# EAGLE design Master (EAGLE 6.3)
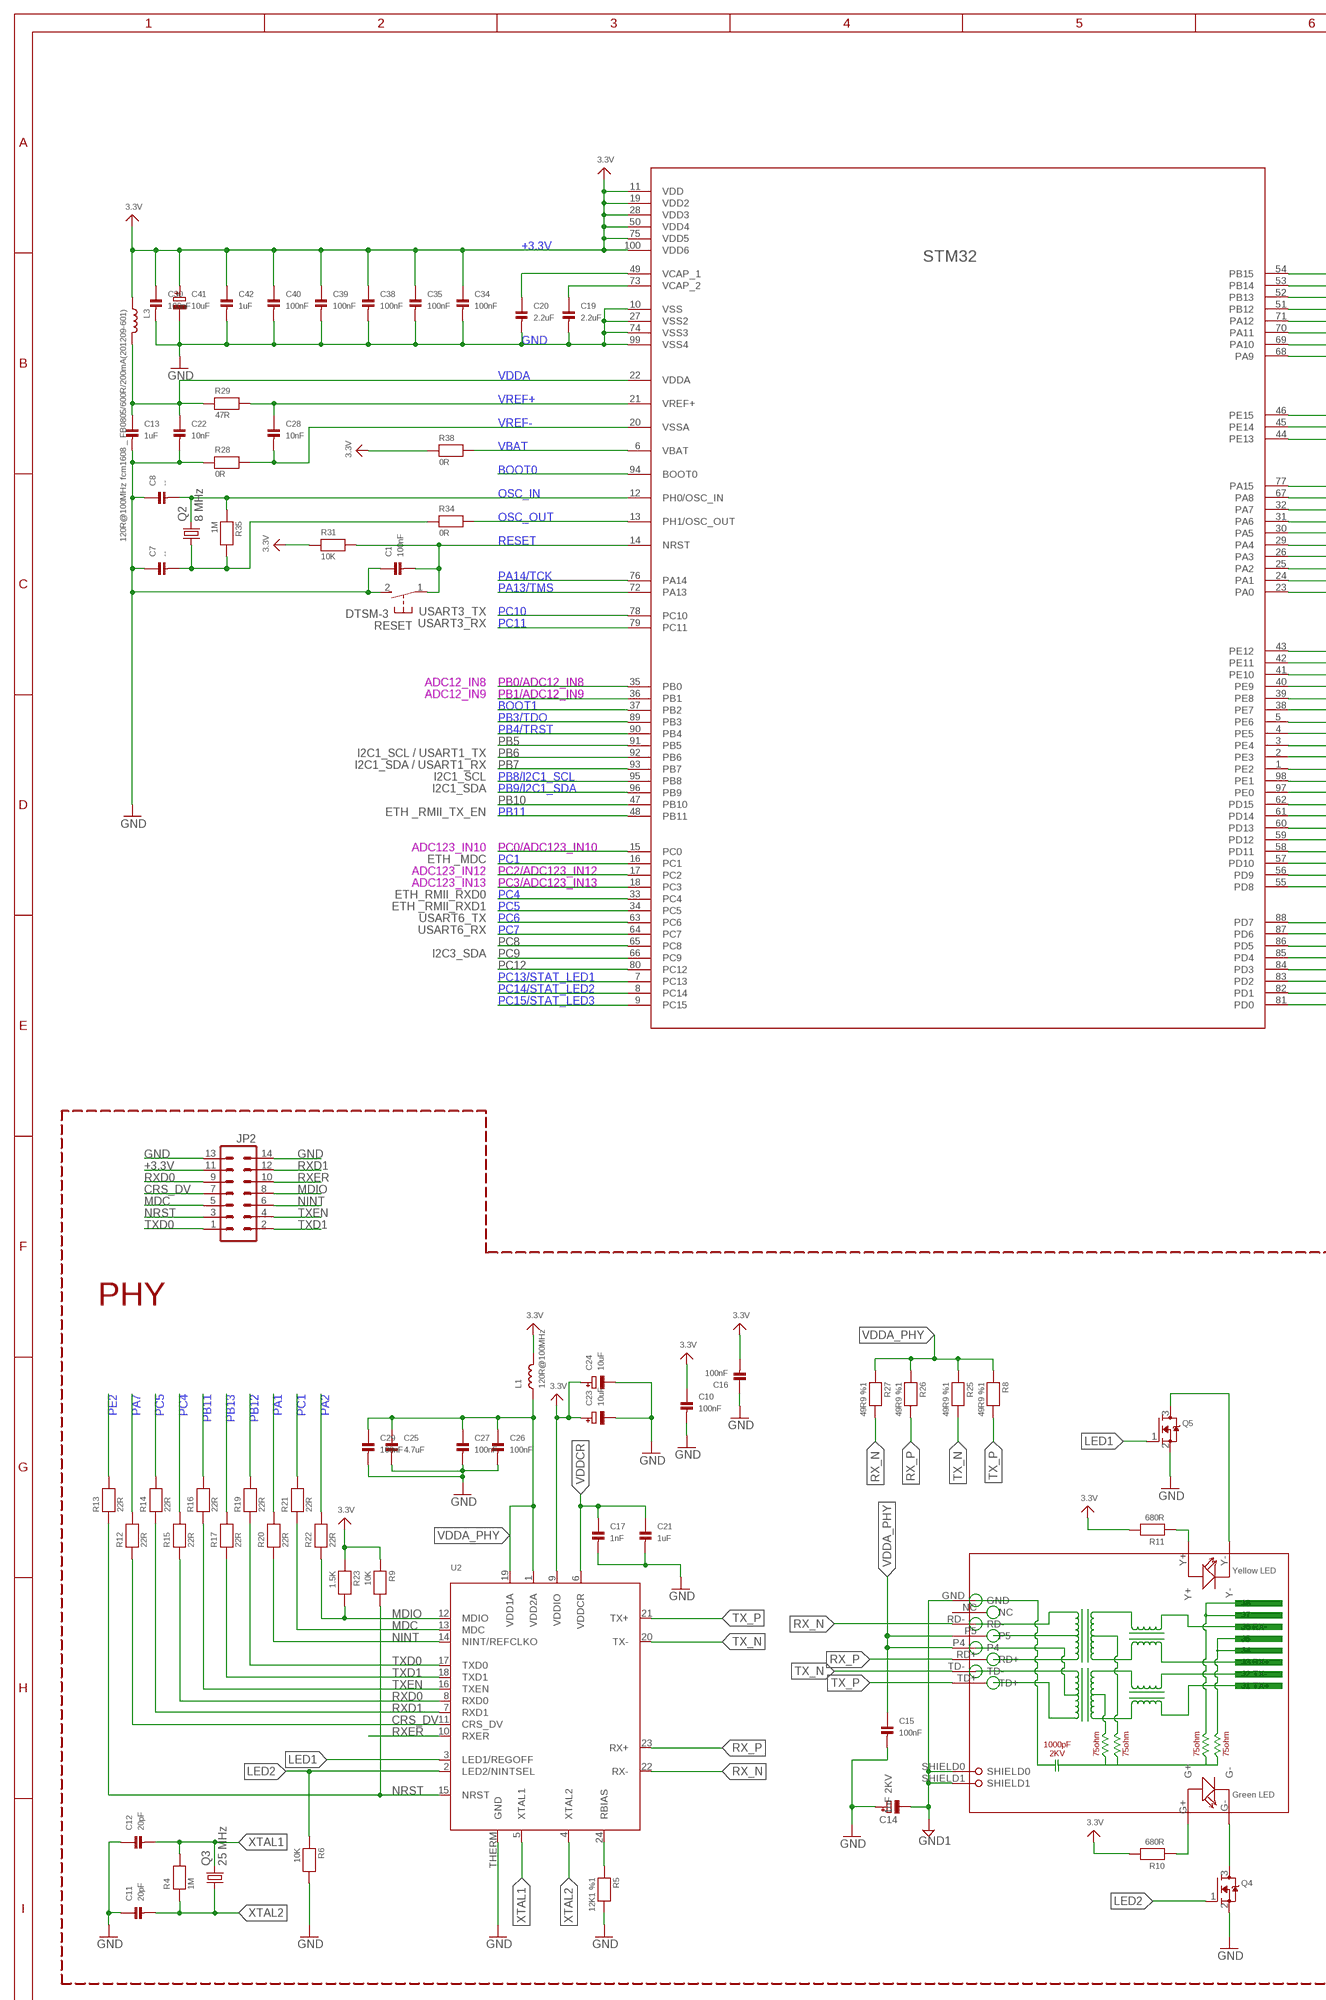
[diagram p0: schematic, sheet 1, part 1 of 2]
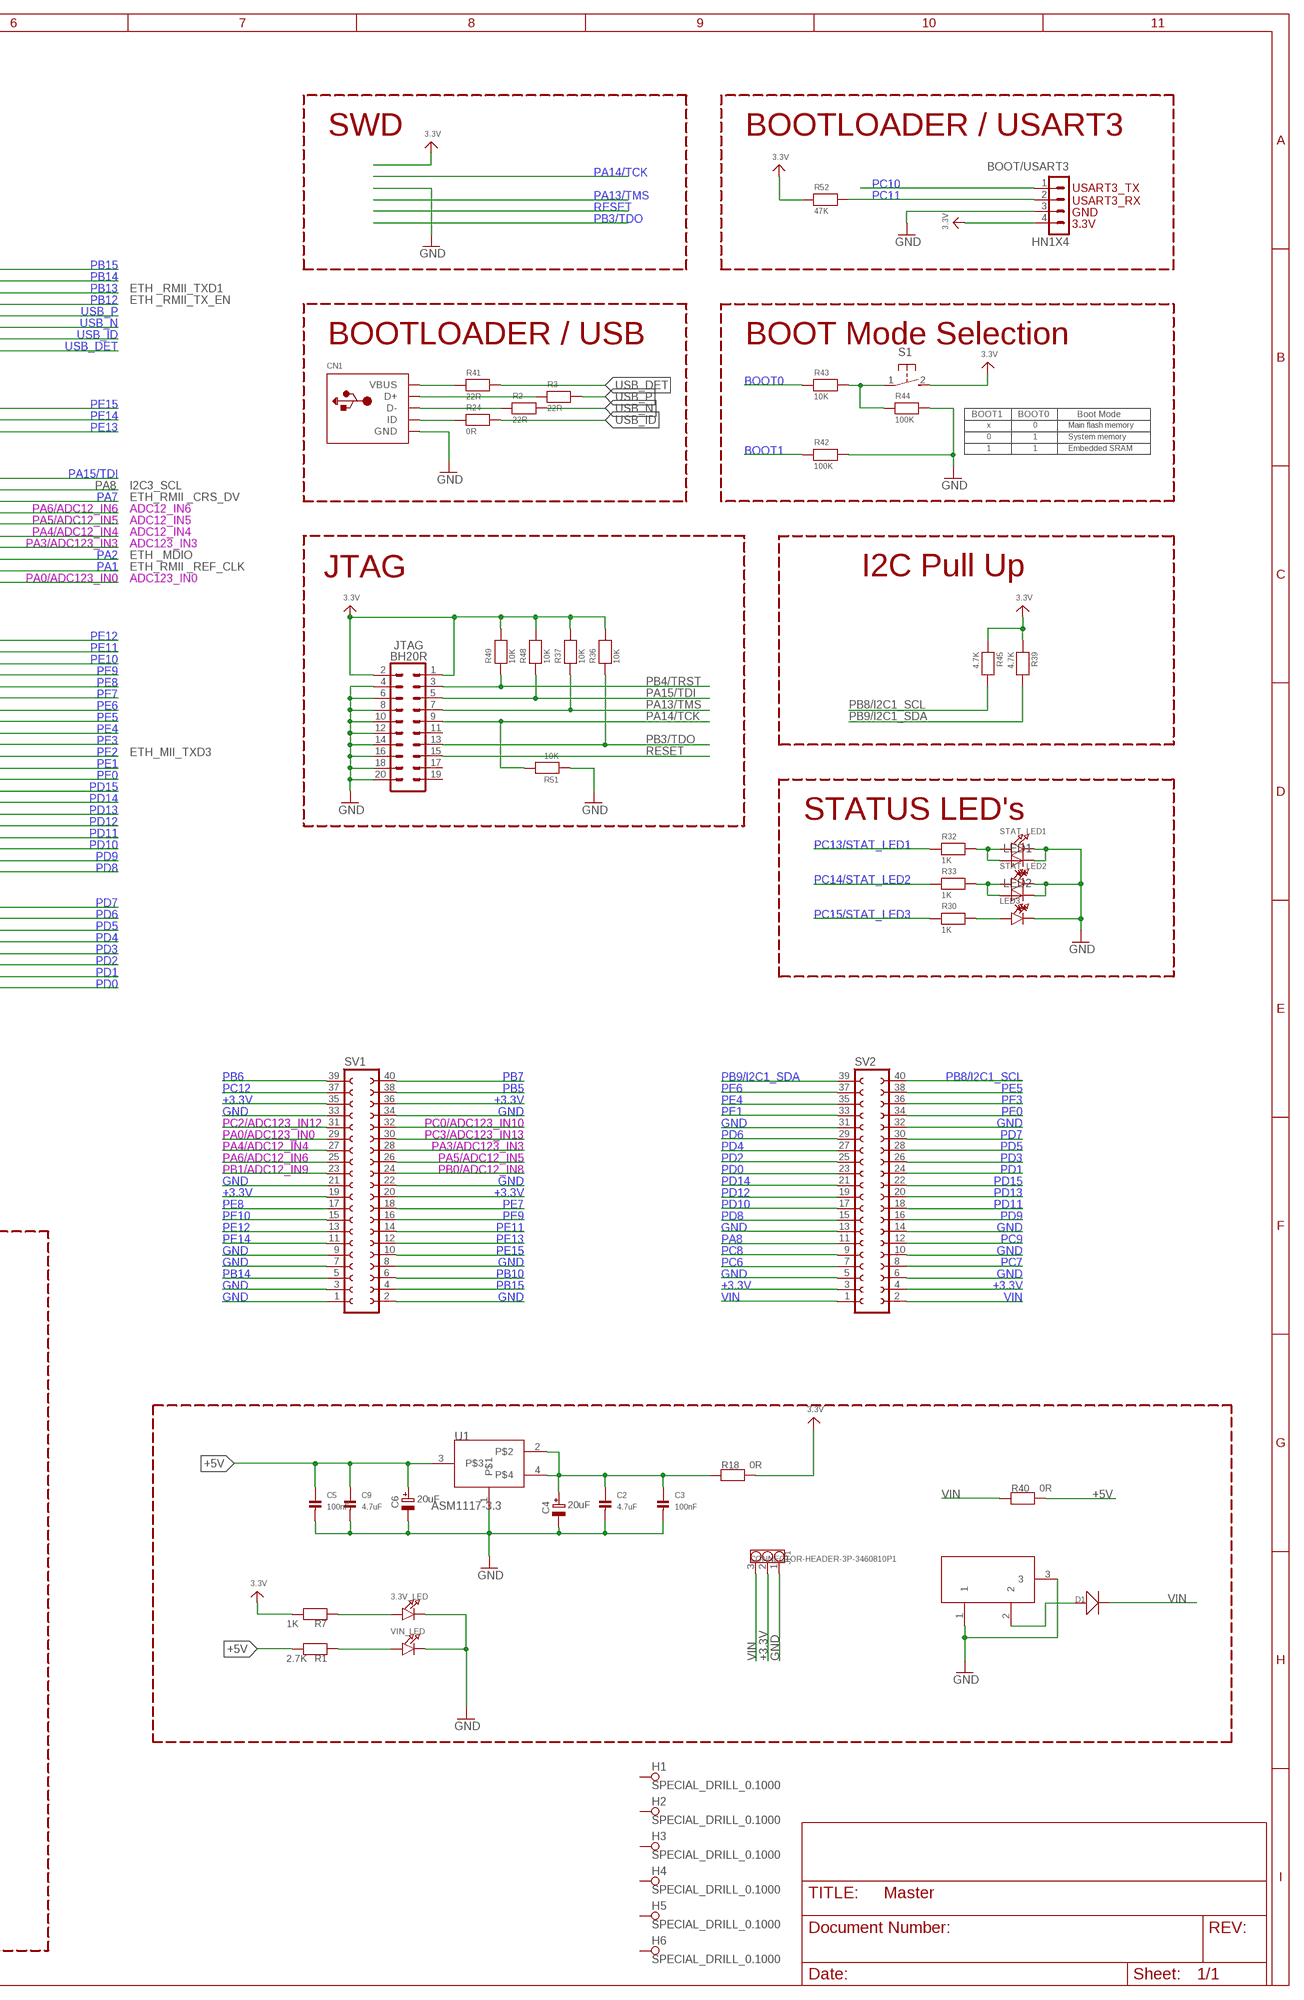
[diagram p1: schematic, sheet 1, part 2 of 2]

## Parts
3.3V_LED  LED0805  [CHIPLED_0805]
BOOT/USART3  HN1X4  CON4HN1X4  [HN1X4]
C1  100nF  CAP_CERAMIC_0603  [_0603]
C2  4.7uF  CAP_CERAMIC0805  [0805]
C3  100nF  CAP_CERAMIC0805  [0805]
C4  20uF  CAP_TANTALUMB/3528_REFLOW  [EIA3528-21/B-R]
C5  100nF  CAP_CERAMIC0805  [0805]
C6  20uF  CAP_TANTALUMB/3528_REFLOW  [EIA3528-21/B-R]
C7  --  CAP_CERAMIC_0603  [_0603]
C8  --  CAP_CERAMIC_0603  [_0603]
C9  4.7uF  CAP_CERAMIC0805  [0805]
C10  100nF  CAP_CERAMIC_0603  [_0603]
C11  20pF  CAP_CERAMIC_0603  [_0603]
C12  20pF  CAP_CERAMIC_0603  [_0603]
C13  1uF  CAP_CERAMIC_0805  [_0805]
C14  1nF 2KV  CAP_TANTALUMB/3528_REFLOW  [EIA3528-21/B-R]
C15  100nF  CAP_CERAMIC_0805  [_0805]
C16  100nF  CAP_CERAMIC_0603  [_0603]
C17  1nF  CAP_CERAMIC_0603  [_0603]
C19  2.2uF  CAP_CERAMIC1206  [1206]
C20  2.2uF  CAP_CERAMIC1206  [1206]
C21  1uF  CAP_CERAMIC_0805  [_0805]
C22  10nF  CAP_CERAMIC_0603  [_0603]
C23  10uF  CAP_TANTALUMB/3528_REFLOW  [EIA3528-21/B-R]
C24  10uF  CAP_TANTALUMB/3528_REFLOW  [EIA3528-21/B-R]
C25  4.7uF  CAP_CERAMIC_0805  [_0805]
C26  100nF  CAP_CERAMIC_0603  [_0603]
C27  100nF  CAP_CERAMIC_0603  [_0603]
C28  10nF  CAP_CERAMIC_0603  [_0603]
C29  100nF  CAP_CERAMIC_0603  [_0603]
C30  100nF  CAP_CERAMIC_0603  [_0603]
C34  100nF  CAP_CERAMIC_0603  [_0603]
C35  100nF  CAP_CERAMIC_0603  [_0603]
C38  100nF  CAP_CERAMIC_0603  [_0603]
C39  100nF  CAP_CERAMIC_0603  [_0603]
C40  100nF  CAP_CERAMIC_0603  [_0603]
C41  10uF  CAP_TANTALUMB/3528_REFLOW  [EIA3528-21/B-R]
C42  1uF  CAP_CERAMIC_0805  [_0805]
CN1  USBMINIBLARGE  [USB-MINIB_LARGER]
D1  D-D1206  [LL-34]
H1  SPECIAL_DRILL_0.1000  [PAD_0.1000]
H2  SPECIAL_DRILL_0.1000  [PAD_0.1000]
H3  SPECIAL_DRILL_0.1000  [PAD_0.1000]
H4  SPECIAL_DRILL_0.1000  [PAD_0.1000]
H5  SPECIAL_DRILL_0.1000  [PAD_0.1000]
H6  SPECIAL_DRILL_0.1000  [PAD_0.1000]
JP1  CONNECTOR-HEADER-3P-3460810P1  [1X3P-2.54-2.54-11.6-3.0-BLACK-MALE]
JP2  MA07-2  [MA07-2]
JTAG  BH20R  ML20R  [BH20R]
L1  120R@100MHz  INDUCTOR_0805  [_0805]
L3  120R@100MHz fcm1608 _ FB0805/600R/200mA(201209-601)  INDUCTOR_0805  [_0805]
LED1  LED5MM  [LED5MM]
LED2  LED5MM  [LED5MM]
LED3  LED0805  [CHIPLED_0805]
Q2  8 MHz  CRYSTALHC49UP  [HC49UP]
Q3  25 MHz  CRYSTALHC49UP  [HC49UP]
Q4  MOSFET-NWIDE  [SOT23-WIDE]
Q5  MOSFET-NWIDE  [SOT23-WIDE]
R1  2.7K  RESISTOR_0603  [_0603]
R2  22R  RESISTOR_0603  [_0603]
R3  22R  RESISTOR_0603  [_0603]
R4  1M  RESISTOR_0603  [_0603]
R5  12K1 %1  RESISTOR_0603  [_0603]
R6  10K  RESISTOR_0603  [_0603]
R7  1K  RESISTOR_0603  [_0603]
R8  49R9 %1  RESISTOR_0603  [_0603]
R9  10K  RESISTOR_0603  [_0603]
R10  680R  RESISTOR_0805  [_0805]
R11  680R  RESISTOR_0805  [_0805]
R12  22R  RESISTOR_0603  [_0603]
R13  22R  RESISTOR_0603  [_0603]
R14  22R  RESISTOR_0603  [_0603]
R15  22R  RESISTOR_0603  [_0603]
R16  22R  RESISTOR_0603  [_0603]
R17  22R  RESISTOR_0603  [_0603]
R18  0R  RESISTOR0805  [0805]
R19  22R  RESISTOR_0603  [_0603]
R20  22R  RESISTOR_0603  [_0603]
R21  22R  RESISTOR_0603  [_0603]
R22  22R  RESISTOR_0603  [_0603]
R23  1.5K  RESISTOR_0603  [_0603]
R24  0R  RESISTOR_0603  [_0603]
R25  49R9 %1  RESISTOR_0603  [_0603]
R26  49R9 %1  RESISTOR_0603  [_0603]
R27  49R9 %1  RESISTOR_0603  [_0603]
R28  0R  RESISTOR_0603  [_0603]
R29  47R  RESISTOR_0603  [_0603]
R30  1K  RESISTOR_0603  [_0603]
R31  10K  RESISTOR_0603  [_0603]
R32  1K  RESISTOR_0603  [_0603]
R33  1K  RESISTOR_0603  [_0603]
R34  0R  RESISTOR_0603  [_0603]
R35  1M  RESISTOR_0603  [_0603]
R36  10K  RESISTOR_0603  [_0603]
R37  10K  RESISTOR_0603  [_0603]
R38  0R  RESISTOR_0603  [_0603]
R39  4.7K  RESISTOR1206  [1206]
R40  0R  RESISTOR0805  [0805]
R41  22R  RESISTOR_0603  [_0603]
R42  100K  RESISTOR_0603  [_0603]
R43  10K  RESISTOR_0603  [_0603]
R44  100K  RESISTOR_0603  [_0603]
R45  4.7K  RESISTOR1206  [1206]
R48  10K  RESISTOR_0603  [_0603]
R49  10K  RESISTOR_0603  [_0603]
R51  10K  RESISTOR_0603  [_0603]
R52  47K  RESISTOR_0603  [_0603]
RESET  DTSM-3  [DTSM-3]
RJ1  HR911105A  [HR911105A]
S1  31-XX  [B3F-31XX]
STAT_LED1  LED0805  [CHIPLED_0805]
STAT_LED2  LED0805  [CHIPLED_0805]
STM32  STM32F407  [100LQFP]
SV1  FE20-2  [FE20-2]
SV2  FE20-2  [FE20-2]
U1  ASM1117-3.3  [SOT223]
U2  LAN8720  [QFN24_4MM]
VIN_LED  LED0805  [CHIPLED_0805]
X1  DC21MMX  [DC-21MM]

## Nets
+3.3V: BOOT/USART3.4 C10.1 C16.2 C23.+ C24.+ C30.1 C34.1 C35.1 C38.1 C39.1 C40.1 C41.+ C42.1 JP1.2 JP2.11 JTAG.1 JTAG.2 L1.2 L3.1 R7.2 R9.1 R10.2 R11.2 R18.2 R23.1 R31.1 R36.2 R37.2 R38.1 R39.1 R45.1 R48.2 R49.2 R52.1 S1.2(S) STM32.11(VDD) STM32.19(VDD2) STM32.28(VDD3) STM32.50(VDD4) STM32.75(VDD5) STM32.100(VDD6) SV1.19 SV1.20 SV1.35 SV1.36 SV2.3 SV2.4 U2.9(VDDIO) ; supply symbol labelled 3.3V
+5V: C5.1 C6.+ C9.1 R1.2 R40.2 U1.3
BOOT0: R43.1 STM32.94(BOOT0)
BOOT1: R42.1 STM32.37(PB2)
CRS_DV: JP2.7 R12.1 U2.11(CRS_DV)
GND: 3.3V_LED.C BOOT/USART3.3 C1.1 C2.2 C3.2 C4.- C5.2 C6.- C7.1 C8.1 C9.2 C10.2 C11.1 C12.1 C13.2 C14.+ C15.2 C16.1 C17.2 C19.2 C20.2 C21.2 C22.2 C23.- C24.- C25.2 C26.2 C27.2 C29.2 C30.2 C34.2 C35.2 C38.2 C39.2 C40.2 C41.- C42.2 CN1.GND JP1.1 JP2.13 JP2.14 JTAG.4 JTAG.6 JTAG.8 JTAG.10 JTAG.12 JTAG.14 JTAG.16 JTAG.18 JTAG.20 LED1.K(C) LED2.K(C) LED3.C Q4.2(S) Q5.2(S) R5.2 R6.2 R28.1 R42.2 R44.2 R51.1 RESET.2 STAT_LED1.C STAT_LED2.C STM32.10(VSS) STM32.27(VSS2) STM32.74(VSS3) STM32.99(VSS4) SV1.1 SV1.2 SV1.3 SV1.7 SV1.8 SV1.9 SV1.21 SV1.22 SV1.33 SV1.34 SV2.5 SV2.6 SV2.10 SV2.13 SV2.14 SV2.31 SV2.32 U1.1 U2.THERM(GND) VIN_LED.C X1.1 X1.3
GND1: C14.- RJ1.GND RJ1.SHIELD0 RJ1.SHIELD1
LED1: Q5.1(G) U2.3(LED1/REGOFF)
LED2: Q4.1(G) R6.1 U2.2(LED2/NINTSEL)
MDC: JP2.5 R21.1 U2.13(MDC)
MDIO: JP2.8 R22.1 R23.2 U2.12(MDIO)
N$1: LED1.A R32.2 STAT_LED1.A
N$2: LED2.A R33.2 STAT_LED2.A
N$3: CN1.VBUS R41.1
N$4: LED3.A R30.2
N$5: D1.A(+) X1.2
N$6: C2.1 C3.1 C4.+ R18.1 U1.2 U1.4
N$7: 3.3V_LED.A R7.1
N$8: R43.2 R44.1 S1.1(P)
N$9: CN1.ID R24.1
N$10: R1.1 VIN_LED.A
N$11: CN1.D+ R3.1
N$12: R5.1 U2.24(RBIAS)
N$13: R10.1 RJ1.G+
N$14: R11.1 RJ1.Y+
N$27: Q4.3(D) RJ1.G-
N$28: Q5.3(D) RJ1.Y-
N$29: CN1.D- R2.1
N$35: C19.1 STM32.73(VCAP_2)
N$36: C20.1 STM32.49(VCAP_1)
N$45: C7.2 Q2.1 R34.1 R35.2
NINT: JP2.6 R20.1 U2.14(NINT/REFCLKO)
NRST: JP2.3 R9.2 R13.1 U2.15(NRST)
OSC_IN: C8.2 Q2.2 R35.1 STM32.12(PH0/OSC_IN)
OSC_OUT: R34.2 STM32.13(PH1/OSC_OUT)
PA0/ADC123_IN0: STM32.23(PA0) SV1.29
PA1: R20.2 STM32.24(PA1)
PA2: R22.2 STM32.25(PA2)
PA3/ADC123_IN3: STM32.26(PA3) SV1.28
PA4/ADC12_IN4: STM32.29(PA4) SV1.27
PA5/ADC12_IN5: STM32.30(PA5) SV1.26
PA6/ADC12_IN6: STM32.31(PA6) SV1.25
PA7: R12.2 STM32.32(PA7)
PA8: STM32.67(PA8) SV2.11
PA13/TMS: JTAG.7 R37.1 STM32.72(PA13)
PA14/TCK: JTAG.9 R51.2 STM32.76(PA14)
PA15/TDI: JTAG.5 R48.1 STM32.77(PA15)
PB0/ADC12_IN8: STM32.35(PB0) SV1.24
PB1/ADC12_IN9: STM32.36(PB1) SV1.23
PB3/TDO: JTAG.13 R36.1 STM32.89(PB3)
PB4/TRST: JTAG.3 R49.1 STM32.90(PB4)
PB5: STM32.91(PB5) SV1.38
PB6: STM32.92(PB6) SV1.39
PB7: STM32.93(PB7) SV1.40
PB8/I2C1_SCL: R45.2 STM32.95(PB8) SV2.40
PB9/I2C1_SDA: R39.2 STM32.96(PB9) SV2.39
PB10: STM32.47(PB10) SV1.6
PB11: R16.2 STM32.48(PB11)
PB12: R19.2 STM32.51(PB12)
PB13: R17.2 STM32.52(PB13)
PB14: STM32.53(PB14) SV1.5
PB15: STM32.54(PB15) SV1.4
PC0/ADC123_IN10: STM32.15(PC0) SV1.32
PC1: R21.2 STM32.16(PC1)
PC2/ADC123_IN12: STM32.17(PC2) SV1.31
PC3/ADC123_IN13: STM32.18(PC3) SV1.30
PC4: R15.2 STM32.33(PC4)
PC5: R14.2 STM32.34(PC5)
PC6: STM32.63(PC6) SV2.7
PC7: STM32.64(PC7) SV2.8
PC8: STM32.65(PC8) SV2.9
PC9: STM32.66(PC9) SV2.12
PC10: BOOT/USART3.1 STM32.78(PC10)
PC11: BOOT/USART3.2 R52.2 STM32.79(PC11)
PC12: STM32.80(PC12) SV1.37
PC13/STAT_LED1: R32.1 STM32.7(PC13)
PC14/STAT_LED2: R33.1 STM32.8(PC14)
PC15/STAT_LED3: R30.1 STM32.9(PC15)
PD0: STM32.81(PD0) SV2.23
PD1: STM32.82(PD1) SV2.24
PD2: STM32.83(PD2) SV2.25
PD3: STM32.84(PD3) SV2.26
PD4: STM32.85(PD4) SV2.27
PD5: STM32.86(PD5) SV2.28
PD6: STM32.87(PD6) SV2.29
PD7: STM32.88(PD7) SV2.30
PD8: STM32.55(PD8) SV2.15
PD9: STM32.56(PD9) SV2.16
PD10: STM32.57(PD10) SV2.17
PD11: STM32.58(PD11) SV2.18
PD12: STM32.59(PD12) SV2.19
PD13: STM32.60(PD13) SV2.20
PD14: STM32.61(PD14) SV2.21
PD15: STM32.62(PD15) SV2.22
PE0: STM32.97(PE0) SV2.34
PE1: STM32.98(PE1) SV2.33
PE2: R13.2 STM32.1(PE2)
PE3: STM32.2(PE3) SV2.36
PE4: STM32.3(PE4) SV2.35
PE5: STM32.4(PE5) SV2.38
PE6: STM32.5(PE6) SV2.37
PE7: STM32.38(PE7) SV1.18
PE8: STM32.39(PE8) SV1.17
PE9: STM32.40(PE9) SV1.16
PE10: STM32.41(PE10) SV1.15
PE11: STM32.42(PE11) SV1.14
PE12: STM32.43(PE12) SV1.13
PE13: STM32.44(PE13) SV1.12
PE14: STM32.45(PE14) SV1.11
PE15: STM32.46(PE15) SV1.10
RESET: C1.2 JTAG.15 R31.2 RESET.1 STM32.14(NRST)
RX_N: R27.2 RJ1.RD- U2.22(RX-)
RX_P: R26.2 RJ1.RD+ U2.23(RX+)
RXD0: JP2.9 R15.1 U2.8(RXD0)
RXD1: JP2.12 R14.1 U2.7(RXD1)
RXER: JP2.10 U2.10(RXER)
TX_N: R25.2 RJ1.TD- U2.20(TX-)
TX_P: R8.2 RJ1.TD+ U2.21(TX+)
TXD0: JP2.1 R19.1 U2.17(TXD0)
TXD1: JP2.2 R17.1 U2.18(TXD1)
TXEN: JP2.4 R16.1 U2.16(TXEN)
USB_DET: R41.2 STM32.68(PA9)
USB_ID: R24.2 STM32.69(PA10)
USB_N: R2.2 STM32.70(PA11)
USB_P: R3.2 STM32.71(PA12)
VBAT: R38.2 STM32.6(VBAT)
VDDA: C13.1 C22.1 L3.2 R29.1 STM32.22(VDDA)
VDDA_PHY: C15.1 C25.1 C26.1 C27.1 C29.1 L1.1 R8.1 R25.1 R26.1 R27.1 RJ1.P4 RJ1.P5 U2.1(VDD2A) U2.19(VDD1A)
VDDCR: C17.1 C21.1 U2.6(VDDCR)
VIN: D1.C(-) JP1.3 R40.1 SV2.1 SV2.2
VREF+: C28.1 R29.2 STM32.21(VREF+)
VREF-: C28.2 R28.2 STM32.20(VSSA)
XTAL1: C12.2 Q3.2 R4.2 U2.5(XTAL1)
XTAL2: C11.2 Q3.1 R4.1 U2.4(XTAL2)
Unconnected: H1.1 H2.1 H3.1 H4.1 H5.1 H6.1 JTAG.11 JTAG.17 JTAG.19 RJ1.NC

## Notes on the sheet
- SWD | BOOTLOADER / USART3
- USART3_TX
- USART3_RX
- GND
- 3.3V
- ETH _RMII_TXD1
- ETH _RMII_TX_EN
- BOOTLOADER / USB | BOOT Mode Selection
- BOOT1 | BOOT0 | Boot Mode
- x | 0 | Main flash memory
- 0 | 1 | System memory
- 1 | 1 | Embedded SRAM
- I2C3_SCL
- ETH_RMII _CRS_DV
- ADC12_IN6
- ADC12_IN5
- ADC12_IN4
- ADC123_IN3
- ETH _MDIO
- ETH_RMII _REF_CLK
- JTAG | I2C Pull Up
- ADC123_IN0
- USART3_TX
- USART3_RX
- ADC12_IN8
- ADC12_IN9
- I2C1_SCL / USART1_TX
- I2C1_SDA / USART1_RX | ETH_MII_TXD3
- I2C1_SCL
- I2C1_SDA
- ETH _RMII_TX_EN
- STATUS LED's
- ADC123_IN10
- ETH _MDC
- ADC123_IN12
- ADC123_IN13
- ETH_RMII_RXD0
- ETH _RMII_RXD1
- USART6_TX
- USART6_RX
- I2C3_SDA
- PHY

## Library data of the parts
3.3V_LED LED3 STAT_LED1 STAT_LED2 VIN_LED = microbuilder:LED: LED
BOOT/USART3 = Penko:CON4
C1-C3 C5 C7-C13 C15-C17 C19-C22 C25-C30 C34 C35 C38-C40 C42 = microbuilder:CAP_CERAMIC: Ceramic Capacitors
C4 C6 C14 C23 C24 C41 = microbuilder:CAP_TANTALUM: Tantalum Capacitors
CN1 = microbuilder:USB: USB Connectors USBMINIB - Surface Mount Female Mini-B USB Connector 4UConnector: 06564
D1 = OPL Eagle Library:D*: DIODE
H1-H6 = special-drill:SPECIAL_DRILL_: Special drills
JP1 = OPL Eagle Library:CONNECTOR-HEADER-3P
JP2 = con-lstb:MA07-2: PIN HEADER; OC_FARNELL: unknown; OC_NEWARK: unknown
JTAG = con-harting-ml:ML20: HARTING
L1 L3 = microbuilder:INDUCTOR: Inductors
LED1 LED2 = led:LED: LED
Q2 Q3 = crystal:CRYSTAL: CRYSTAL; OC_FARNELL: unknown; OC_NEWARK: unknown
Q4 Q5 = microbuilder:MOSFET-N: N-Channel Mosfet LEGEND VDS: Voltage Drain-Source ID: Drain Current RDS(ON): Drain-Source On-State Resistance VGS(TH): Gate-Source Threshold Voltage CISS: Drain-Source Input Capacitance SOT-23 Name VDS ID RDS(ON) VGS(TH) CISS Order Number 2N7002E 60V 260mA 2.5 Ohm 2.5V @ 250uA 26.7pF @ 25V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
R1-R45 R48 R49 R51 R52 = microbuilder:RESISTOR: Resistors
RESET = switch-tact:DTSM-3
RJ1 = Itead_BP_110825.lbr:HR911105A: SOC006
S1 = switch-omron:31-XX: OMRON SWITCH; MPN: B3F-3100; OC_FARNELL: 959704; OC_NEWARK: 36M3582
STM32 = BaseApp:STM32F407
SV1 SV2 = con-lsta:FE20-2: FEMALE HEADER; OC_FARNELL: unknown; OC_NEWARK: unknown
U1 = Itead_IC_110429:ASM1117-3.3: ICP006
U2 = microbuilder:LAN8720: LAN8720A 10/100 Ethernet PHY Mouser: 886-LAN8720AI-CP
X1 = powersupply:DC21MM

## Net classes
0 default: width 0.152 mm, drill 0.305 mm, clearance 0.152 mm

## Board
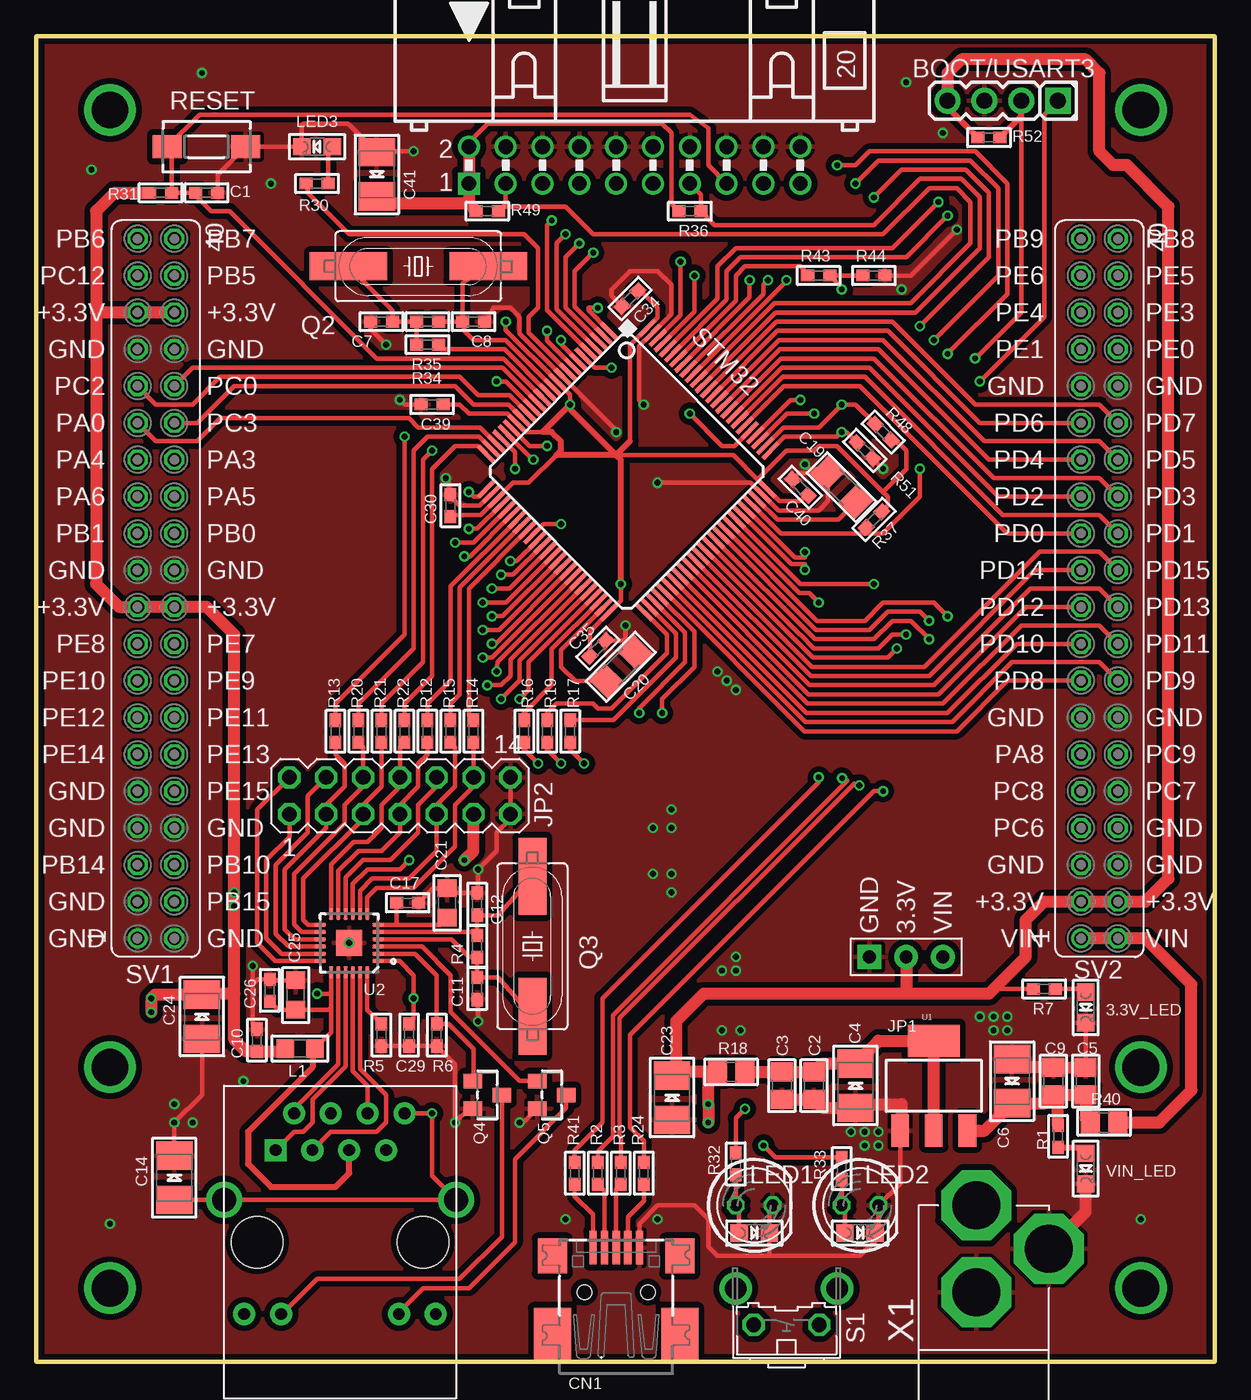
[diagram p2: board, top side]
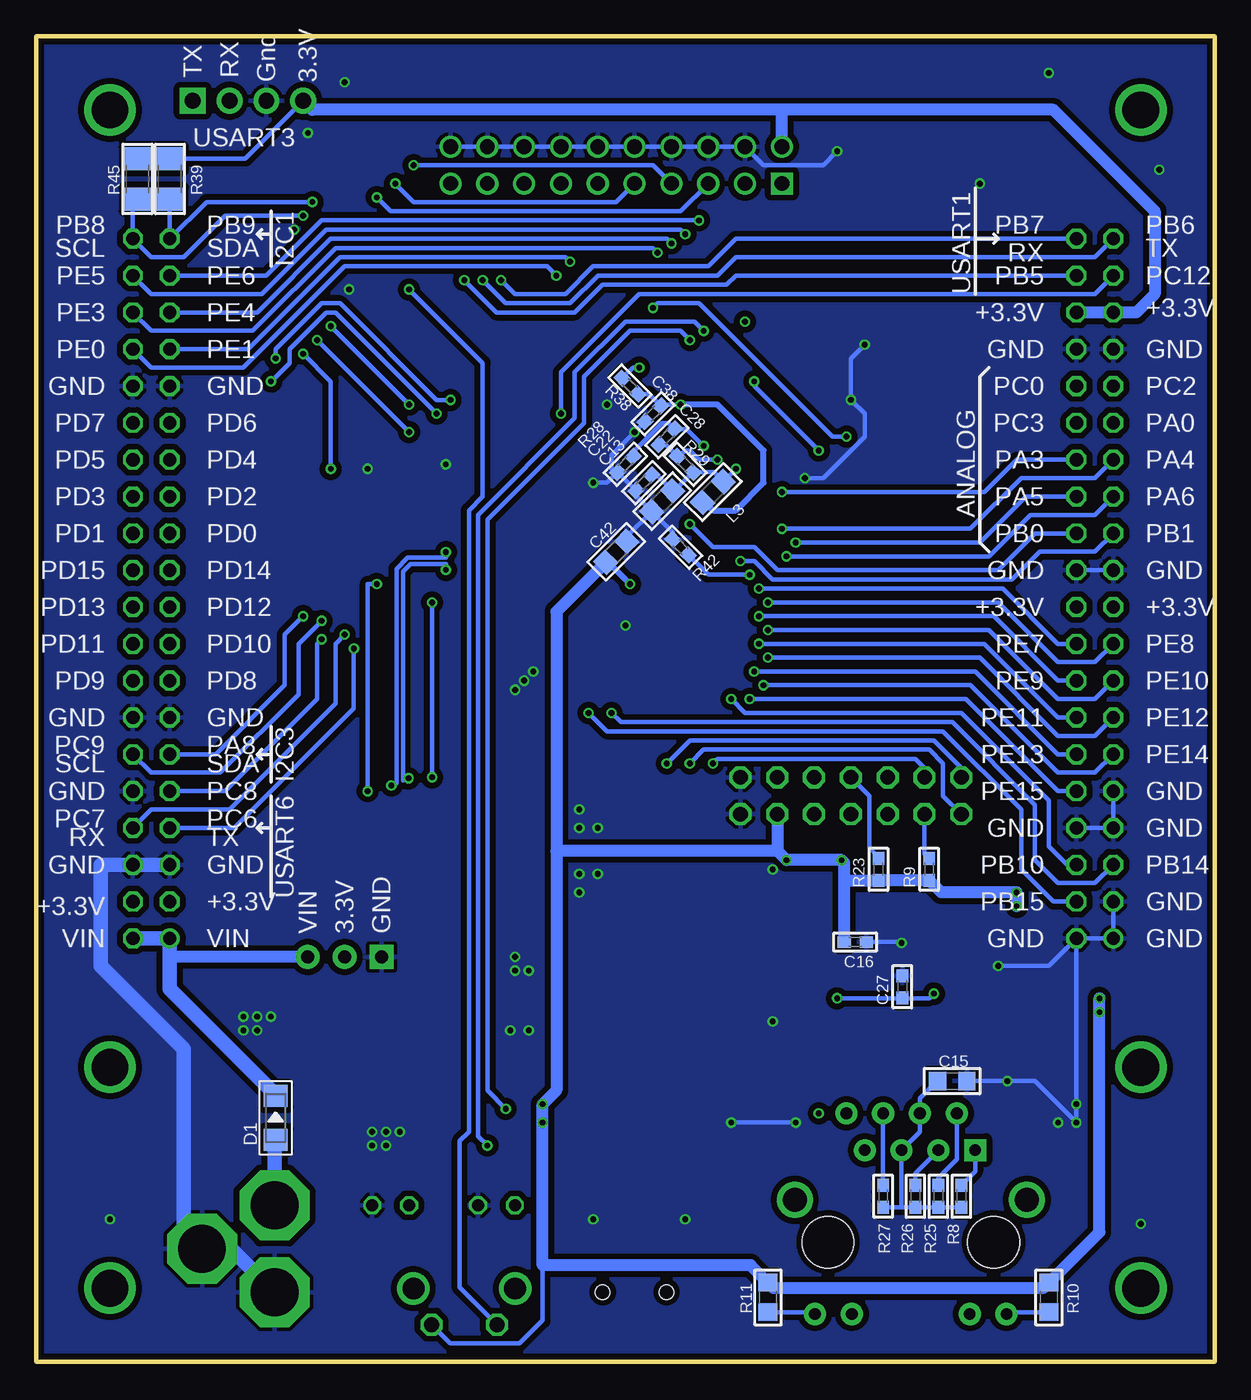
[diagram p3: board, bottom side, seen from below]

Size 81.28 x 91.44 mm. Coordinates in mm from the lower left corner, seen from the top.
Outline: 0,0 81.28,0 81.28,91.44 0,91.44 0,0
Copper layers (1*2*15*16): Top 0.035mm / dielectric 0.2mm / Route2 0.0175mm / dielectric 1.1mm / Route15 0.0175mm / dielectric 0.2mm / Bottom 0.035mm
Design rules "SeeedStudio_DRU_no_angle_20130527": minimum track width 6mil, minimum drill 12mil, track to track 6mil, track to pad 6mil, pad to pad 6mil, via to via 6mil, smd to smd 0mil, copper to edge 10mil, drill to drill 10mil, minimum pad ring 6mil, minimum via ring 6mil, stop-mask expansion 2mil, vias tented up to drill 25mil, thermal gap 10mil

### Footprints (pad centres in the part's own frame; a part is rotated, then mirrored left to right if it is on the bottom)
CHIPLED_0805 = smd 1.2 x 1.2: A 0,-1.05; C 0,1.05
HN1X4 = drill 1.1 pad 1.778 square: 1 -3.81,0 | drill 1.1 pad 1.778: 2 -1.27,0; 3 1.27,0; 4 3.81,0
_0603 = smd 0.9 x 0.8: 1 -0.762,0; 2 0.762,0
0805 = smd 1.3 x 1.5: 1 -0.95,0; 2 0.95,0
EIA3528-21/B-R = smd 1.95 x 2.5: + 1.525,0; - -1.525,0
_0805 = smd 1.2 x 1.3: 1 -1.016,0; 2 1.016,0
1206 = smd 1.6 x 1.8: 1 -1.4,0; 2 1.4,0
USB-MINIB_LARGER = smd 0.5 x 2.308: D+ 0,4.064; D- -0.8,4.064; GND 1.6,4.064; ID 0.8,4.064; VBUS -1.6,4.064 | smd 2.54 x 3.81: GND1 -4.4,-2; GND4 4.4,-2 | smd 2 x 2.4: GND2 -4.4,3.5; GND3 4.4,3.5 | hole 1: -2.2,1; 2.2,1
LL-34 = smd 1.524 x 1.676: A -1.524,0; C 1.524,0
PAD_0.1000 = drill 2.54 pad 2.54: 1 0,0
1X3P-2.54-2.54-11.6-3.0-BLACK-MALE = drill 0.889 pad 1.651 square: 1 0,2.54 | drill 0.889 pad 1.651: 2 0,0; 3 0,-2.54
MA07-2 = drill 1.016 octagon: 1 -7.62,-1.27; 2 -7.62,1.27; 3 -5.08,-1.27; 4 -5.08,1.27; 5 -2.54,-1.27; 6 -2.54,1.27; 7 0,-1.27; 8 0,1.27; 9 2.54,-1.27; 10 2.54,1.27; 11 5.08,-1.27; 12 5.08,1.27; 13 7.62,-1.27; 14 7.62,1.27
BH20R = drill 1.016 square: 1 -11.43,-1.27 | drill 1.016: 2 -11.43,1.27; 3 -8.89,-1.27; 4 -8.89,1.27; 5 -6.35,-1.27; 6 -6.35,1.27; 7 -3.81,-1.27; 8 -3.81,1.27; 9 -1.27,-1.27; 10 -1.27,1.27; 11 1.27,-1.27; 12 1.27,1.27; 13 3.81,-1.27; 14 3.81,1.27; 15 6.35,-1.27; 16 6.35,1.27; 17 8.89,-1.27; 18 8.89,1.27; 19 11.43,-1.27; 20 11.43,1.27
LED5MM = drill 0.813 octagon: A -1.27,0; K 1.27,0
HC49UP = smd 5.334 x 1.93: 1 -4.826,0; 2 4.826,0
SOT23-WIDE = smd 1 x 1.27: 1 -0.95,-1; 2 0.95,-1; 3 0,1
DTSM-3 = smd 2 x 1.6: 1 -2.7,0; 2 2.7,0
HR911105A = drill 0.813 pad 1.524: G+ 4.953,-6.604; G- 4.953,-4.064; GND -8.89,4.445; NC -6.35,3.175; P4 -8.89,-0.635; P5 -6.35,0.635; RD+ -6.35,-1.905; RD- -8.89,1.905; TD- -8.89,-3.175; Y+ 4.953,6.604; Y- 4.953,4.064 | drill 1.651 pad 2.159: SHIELD0 -2.921,8.001; SHIELD1 -2.921,-8.001 | drill 0.813 pad 1.524 square: TD+ -6.35,-4.445 | hole 3.556: 0,-5.715; 0,5.715
B3F-31XX = drill 1.016 octagon: 1 -2.261,-1.245; 2 2.261,-1.245 | drill 1.499 pad 2.159: 3 -3.505,1.245; 4 3.505,1.245
100LQFP = smd 1.5 x 0.3: 1 -6.18,9.08; 2 -6.18,8.58; 3 -6.18,8.08; 4 -6.18,7.58; 5 -6.18,7.08; 6 -6.18,6.58; 7 -6.18,6.08; 8 -6.18,5.58; 9 -6.18,5.08; 10 -6.18,4.58; 11 -6.18,4.08; 12 -6.18,3.58; 13 -6.18,3.08; 14 -6.18,2.58; 15 -6.18,2.08; 16 -6.18,1.58; 17 -6.18,1.08; 18 -6.18,0.58; 19 -6.18,0.08; 20 -6.18,-0.42; 21 -6.18,-0.92; 22 -6.18,-1.42; 23 -6.18,-1.92; 24 -6.18,-2.42; 25 -6.18,-2.92; 51 9.26,-2.92; 52 9.26,-2.42; 53 9.26,-1.92; 54 9.26,-1.42; 55 9.26,-0.92; 56 9.26,-0.42; 57 9.26,0.08; 58 9.26,0.58; 59 9.26,1.08; 60 9.26,1.58; 61 9.26,2.08; 62 9.26,2.58; 63 9.26,3.08; 64 9.26,3.58; 65 9.26,4.08; 66 9.26,4.58; 67 9.26,5.08; 68 9.26,5.58; 69 9.26,6.08; 70 9.26,6.58; 71 9.26,7.08; 72 9.26,7.58; 73 9.26,8.08; 74 9.26,8.58; 75 9.26,9.08 | smd 0.3 x 1.5: 26 -4.46,-4.64; 27 -3.96,-4.64; 28 -3.46,-4.64; 29 -2.96,-4.64; 30 -2.46,-4.64; 31 -1.96,-4.64; 32 -1.46,-4.64; 33 -0.96,-4.64; 34 -0.46,-4.64; 35 0.04,-4.64; 36 0.54,-4.64; 37 1.04,-4.64; 38 1.54,-4.64; 39 2.04,-4.64; 40 2.54,-4.64; 41 3.04,-4.64; 42 3.54,-4.64; 43 4.04,-4.64; 44 4.54,-4.64; 45 5.04,-4.64; 46 5.54,-4.64; 47 6.04,-4.64; 48 6.54,-4.64; 49 7.04,-4.64; 50 7.54,-4.64; 76 7.54,11.1; 77 7.04,11.1; 78 6.54,11.1; 79 6.04,11.1; 80 5.54,11.1; 81 5.04,11.1; 82 4.54,11.1; 83 4.04,11.1; 84 3.54,11.1; 85 3.04,11.1; 86 2.54,11.1; 87 2.04,11.1; 88 1.54,11.1; 89 1.04,11.1; 90 0.54,11.1; 91 0.04,11.1; 92 -0.46,11.1; 93 -0.96,11.1; 94 -1.46,11.1; 95 -1.96,11.1; 96 -2.46,11.1; 97 -2.96,11.1; 98 -3.46,11.1; 99 -3.96,11.1; 100 -4.46,11.1
FE20-2 = drill 0.914: 1 -24.13,1.27 | drill 0.914 octagon: 2 -24.13,-1.27; 3 -21.59,1.27; 4 -21.59,-1.27; 5 -19.05,1.27; 6 -19.05,-1.27; 7 -16.51,1.27; 8 -16.51,-1.27; 9 -13.97,1.27; 10 -13.97,-1.27; 11 -11.43,1.27; 12 -11.43,-1.27; 13 -8.89,1.27; 14 -8.89,-1.27; 15 -6.35,1.27; 16 -6.35,-1.27; 17 -3.81,1.27; 18 -3.81,-1.27; 19 -1.27,1.27; 20 -1.27,-1.27; 21 1.27,1.27; 22 1.27,-1.27; 23 3.81,1.27; 24 3.81,-1.27; 25 6.35,1.27; 26 6.35,-1.27; 27 8.89,1.27; 28 8.89,-1.27; 29 11.43,1.27; 30 11.43,-1.27; 31 13.97,1.27; 32 13.97,-1.27; 33 16.51,1.27; 34 16.51,-1.27; 35 19.05,1.27; 36 19.05,-1.27; 37 21.59,1.27; 38 21.59,-1.27; 39 24.13,1.27; 40 24.13,-1.27
SOT223 = smd 1.219 x 2.235: 1 -2.311,-3.099; 2 0,-3.099; 3 2.311,-3.099 | smd 3.6 x 2.2: 4 0,3.099
QFN24_4MM = smd 0.8 x 0.28: 1 -2,1.25; 2 -2,0.75; 3 -2,0.25; 4 -2,-0.25; 5 -2,-0.75; 6 -2,-1.25; 13 2,-1.25; 14 2,-0.75; 15 2,-0.25; 16 2,0.25; 17 2,0.75; 18 2,1.25 | smd 0.28 x 0.8: 7 -1.25,-2; 8 -0.75,-2; 9 -0.25,-2; 10 0.25,-2; 11 0.75,-2; 12 1.25,-2; 19 1.25,2; 20 0.75,2; 21 0.25,2; 22 -0.25,2; 23 -0.75,2; 24 -1.25,2 | smd 1.778 x 1.778: THERM 0,0
DC-21MM = drill 3.302 pad 4.826 octagon: 1 -5.08,-3.353; 2 -0.076,-6.35; 3 -0.076,-0.356

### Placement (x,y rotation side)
3.3V_LED  72.39,24.45 180 top
BOOT/USART3  66.67,87 180 top
C1  11.75,80.64 180 top
C2  53.66,19.05 270 top
C3  51.44,19.05 270 top
C4  56.52,19.05 90 top
C5  72.39,19.37 90 top
C6  67.31,19.37 270 top
C7  23.81,71.75 0 top
C8  30.16,71.75 180 top
C9  70.17,19.37 90 top
C10  15.22,22.19 90 top
C11  30.41,25.75 90 top
C12  30.41,31.57 270 top
C13  38.1,59.37 225 bottom
C14  9.53,12.7 90 top
C15  18.1,19.37 0 bottom
C16  24.79,28.96 180 bottom
C17  25.62,31.67 0 top
C19  55.56,60.33 135 top
C20  40.32,47.94 45 top
C21  28.34,31.65 90 top
C22  39.37,60.64 225 bottom
C23  43.86,18.23 90 top
C24  11.43,23.81 90 top
C25  17.9,25.3 90 top
C26  16.11,25.62 90 top
C27  21.54,25.87 90 bottom
C28  37.78,63.82 45 bottom
C29  25.72,22.54 270 top
C30  28.57,59.05 90 top
C34  40.96,73.34 225 top
C35  38.73,49.21 45 top
C38  38.73,65.41 225 bottom
C39  27.3,66.04 180 top
C40  52.7,60.33 135 top
C41  23.5,81.92 270 top
C42  41.27,55.88 45 bottom
CN1  40.01,3.81 0 top
D1  64.77,16.83 90 bottom
H1  5.08,5.08 0 top
H2  76.2,5.08 0 top
H3  76.2,86.36 0 top
H4  5.08,86.36 0 top
H5  5.08,20.32 0 top
H6  76.2,20.32 0 top
JP1  60.01,27.94 90 top
JP2  25.08,39.05 0 top
JTAG  41.27,82.55 0 top
L1  18.19,21.61 180 top
L3  34.61,60.01 45 bottom
LED1  49.53,10.79 0 top
LED2  56.83,10.79 0 top
LED3  19.37,83.82 90 top
Q2  26.35,75.56 0 top
Q3  34.22,28.66 90 top
Q4  31.11,18.41 270 top
Q5  35.56,18.41 270 top
R1  70.48,15.56 90 top
R2  38.73,13.02 90 top
R3  40.32,13.02 90 top
R4  30.41,28.66 90 top
R5  23.81,22.54 270 top
R6  27.62,22.54 270 top
R7  69.53,25.72 180 top
R8  17.46,11.43 90 bottom
R9  19.68,33.97 90 bottom
R10  11.43,4.45 90 bottom
R11  30.8,4.45 90 bottom
R12  26.99,43.5 90 top
R13  20.64,43.5 90 top
R14  30.16,43.5 90 top
R15  28.57,43.5 90 top
R16  33.66,43.5 90 top
R17  36.83,43.5 90 top
R18  47.94,20 180 top
R19  35.24,43.5 90 top
R20  22.23,43.5 90 top
R21  23.81,43.5 90 top
R22  25.4,43.5 90 top
R23  23.18,33.97 90 bottom
R24  41.91,13.02 90 top
R25  19.05,11.43 90 bottom
R26  20.64,11.43 90 bottom
R27  22.86,11.43 90 bottom
R28  40.64,61.91 45 bottom
R29  36.51,61.91 135 bottom
R30  19.37,81.28 0 top
R31  8.57,80.64 0 top
R32  48.26,13.65 270 top
R33  55.56,13.34 270 top
R34  26.99,70.17 0 top
R35  26.99,71.75 180 top
R36  45.09,79.38 180 top
R37  57.78,58.1 45 top
R38  40.32,67.31 135 bottom
R39  72.07,81.6 270 bottom
R40  73.66,16.51 180 top
R41  37.15,13.02 90 top
R42  36.83,56.2 135 bottom
R43  53.98,74.93 0 top
R44  57.78,74.93 0 top
R45  74.3,81.6 270 bottom
R48  58.42,64.14 315 top
R49  31.11,79.38 180 top
R51  57.15,62.87 135 top
R52  65.72,84.45 0 top
RESET  11.75,83.82 0 top
RJ1  20.95,8.26 270 top
S1  51.75,3.81 0 top
STAT_LED1  49.53,8.89 270 top
STAT_LED2  56.83,8.89 270 top
STM32  37.47,60.33 315 top
SV1  8.26,53.34 90 top
SV2  73.34,53.34 90 top
U1  61.91,19.05 0 top
U2  21.59,28.89 180 top
VIN_LED  72.39,13.34 180 top
X1  64.77,4.45 180 top

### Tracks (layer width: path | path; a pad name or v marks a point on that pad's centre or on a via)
+3.3V  (via drill 0.4)
  Top 0.305: U2.9 21.84,32.95 22.86,33.97 25.08,33.97 v25.72,34.61 | R36.2 43.81,79.88 43.81,84.77 43.18,85.41 31.11,85.41 29.84,84.14 JTAG.2 | v32.38,71.75 32.38,71.17 STM32.11 36.83,66.73 v36.83,66.04 | 44.13,20.02 C23.+ | R7.2 66.36,25.72 66.2,25.88 | C35.1 38.2,50.39 STM32.50 40.32,52.52 v40.32,53.66 | C30.1 28.45,58.29 28.57,58.42 30.67,58.42 STM32.28 32.89,60.64 33.97,60.64 35.88,62.55 | C39.1 29.21,66.04 29.84,65.41 32.5,65.41 STM32.19 33.77,64.14 34.92,64.14 | C34.1 41.69,73.88 42.86,72.71 42.86,72.03 STM32.100 40.96,70.12 40.96,63.5 | C40.1 53.24,59.91 52.7,59.37 51.26,59.37 STM32.75 49.76,60.87 | R37.2 58.74,59.05 58.74,59.69 58.42,60.01 | 58.42,60.01 55.24,63.18 53.98,63.18 53.66,62.87 51.75,62.87 49.76,60.87 | R48.2 59.59,63.28 60.01,62.87 60.01,61.59 58.42,60.01 | 49.76,60.87 48.08,62.55 40.01,62.55 | 11.49,25.4 C24.+ | 62.87,87.44 BOOT/USART3.4
  Top 0.406: 40.96,63.5 40.01,62.55 | 40.01,62.55 35.88,62.55 36.2,62.87 36.2,63.5 35.56,64.14 34.92,64.14 v36.83,66.04 36.83,65.72 40.01,62.55 | v40.32,53.66 40.32,62.23 40.01,62.55 | R52.1 62.87,86.55 BOOT/USART3.4
  Top 0.813: v29.53,34.61 30.16,35.24 JP2.11 | 29.84,79.88 JTAG.1 JTAG.2 | 29.84,79.88 R49.2 | 60.01,25.4 65.72,25.4 66.2,25.88 68.26,27.94 68.26,30.48 69.53,31.75 SV2.3 SV2.4 76.52,31.75 78.11,33.34 78.11,79.69 75.25,82.55 74.3,82.55 73.34,83.5 73.34,88.9 72.39,89.85 63.82,89.85 62.87,88.9 BOOT/USART3.4 | 60.01,25.4 46.04,25.4 44.13,23.5 44.13,20.02 46.35,20.02 | 46.35,20.02 46.97,20.02 R18.2 | 13.65,25.4 13.65,22.23 14.45,21.43 C10.1 16.99,21.43 L1.2 | 13.65,25.4 11.49,25.4 | 46.35,20.02 v46.35,17.78 v46.35,16.51 | JP1.2 60.01,25.4 | C24.+ 8.19,25.34 v7.94,25.08 v7.94,24.13 | 13.65,25.4 v13.65,32.38 13.65,50.16 11.75,52.07 SV1.20 SV1.19 5.71,52.07 4.13,53.66 4.13,72.39 | SV1.36 SV1.35 4.13,72.39 | 4.13,72.39 4.13,79.38 5.4,80.64 R31.1 | 29.84,79.88 24,79.88 C41.+
  Bottom 0.305: v25.72,34.61 25.55,34.44 | R23.1 23.15,33.34 | 41.83,55.16 C42.1 | v36.83,66.04 38.1,66.04 C38.1 39.02,66.77 R38.1 | S1.2 52.72,1.27 47.94,1.27 46.35,2.86 46.35,6.67 | BOOT/USART3.4 66.86,83 R39.1 R45.1
  Bottom 0.406: v40.32,53.66 41.83,55.16 | L3.1 35.16,59.29 34.61,58.74 33.02,58.74 31.11,60.64 31.11,62.87 34.29,66.04 v36.83,66.04
  Bottom 0.813: v25.72,34.61 v29.53,34.61 30.16,35.24 | 25.55,34.44 25.55,33.34 | 25.55,33.34 C16.2 | v7.94,25.08 7.94,8.95 R10.2 11.81,5.08 30.42,5.08 R11.2 32,6.67 46.35,6.67 v46.35,17.78 45.4,18.73 45.4,35.24 | 25.55,33.34 25.42,33.21 R23.1 R9.1 18.86,32.38 v13.65,32.38 v13.65,31.43 | JP2.11 30.16,35.24 | C42.1 45.4,51.75 45.4,35.24 | 30.16,35.24 45.4,35.24 | SV1.36 SV1.35 5.4,72.39 4.13,73.66 4.13,79.38 11.11,86.36 29.84,86.36 | 29.84,86.36 62.23,86.36 BOOT/USART3.4 | JTAG.2 29.84,86.36
+5V
  Top 0.813: C9.1 C5.1 72.39,16.83 R40.2 | 65.01,15.95 U1.3 65.42,15.95 C6.+ 69.59,17.84 C9.1 | R1.2 70.48,18.1 C9.1
BOOT0
  Top 0.305: STM32.94 48.26,73.19 48.26,74.93 48.9,75.56 52.7,75.56 53.21,75.06 R43.1
BOOT1  (via drill 0.4)
  Top 0.305: STM32.37 32.9,54.29 v32.07,54.29
  Bottom 0.305: v32.07,54.29 34.92,54.29 36.51,55.88 | 36.51,55.88 | 36.51,55.88 R42.1
CRS_DV
  Top 0.305: U2.11 20.84,33.86 22.23,35.24 23.81,35.24 25.08,36.51 JP2.7 25.08,38.42 26.35,39.69 26.35,41.27 26.99,41.91 R12.1
GND  (via drill 0.4)
  Top 0.305: C5.2 3.3V_LED.C | 72.53,10.48 72.39,10.34 | 67.89,20.32 C6.- | 59.69,16.04 U1.1 59.6,12.29 LED2.K 58.1,9.11 STAT_LED2.C 57.88,8.35 56.83,7.3 50.58,7.3 | C4.- 56.77,17.78 | C7.1 23.05,71.25 v24.13,70.17 | C8.1 31.56,72.71 32.7,72.71 33.34,72.07 33.34,70.93 STM32.10 40.01,64.26 v40.01,64.14 | C1.1 12.51,81.88 RESET.2 LED3.C 18.32,85.31 18.41,85.41 21.53,85.41 C41.- 23.56,83.5 v26.04,83.5 | 40.64,49.6 40.48,49.77 39.29,49.77 C35.2 | C20.2 40.64,49.6 | C17.2 27.38,32.67 C21.2 28.67,32.34 C12.1 30.48,32.4 v30.48,33.97 31.75,35.24 31.75,36.51 32.7,37.47 JP2.13 JP2.14 | C25.2 16.17,26.32 C26.2 15.27,26.38 14.92,26.04 | 14.92,26.04 14.92,23.25 C10.2 | R5.2 C29.2 R6.2 28.89,20.51 v28.89,16.51 29.85,17.46 Q4.2 | 40.64,49.6 v40.64,50.8 | STM32.27 30.59,59.05 29.21,59.05 28.45,59.82 | 28.45,59.82 C30.2 | C39.2 25.4,66.04 v25.08,66.36 | 28.45,59.82 28.45,60.77 v28.26,60.96 | v42.86,60.64 49.28,60.64 STM32.74 51.19,58.74 53.98,58.74 54.61,59.37 54.61,61.59 | 54.61,61.59 arc90 C19.2 52.62,61.31 C40.2 | 54.61,61.59 53.34,61.59 v53.02,61.91 | v41.91,66.04 41.59,66.36 41.59,70.05 STM32.99 43.81,72.28 43.81,74.3 42.86,75.25 40.96,75.25 39.69,73.98 39.69,73.53 C34.2 | C14.+ v9.53,16.51 11.43,18.41 C24.- | Q5.2 33.6,16.51 v33.34,16.51 | C11.1 30.48,24.92 v30.48,23.5 | 14.92,26.04 v14.92,27.3 | LED1.K 50.58,10.57 STAT_LED1.C 50.58,7.3 | CN1.GND 41.6,9.54 42.86,10.79 45.4,10.79 46.35,9.84 46.35,7.94 46.99,7.3 50.58,7.3 | R44.2 60.33,74.93 v63.5,78.11 | R51.1 | R51.1 v58.42,61.59
  Top 0.813: X1.1 72.39,10.34 VIN_LED.C | C5.2 C9.2 67.89,20.32 | 59.69,16.04 59.69,17.78 56.77,17.78 | C3.2 C2.2 54.23,17.52 C4.-
  Bottom 0.305: JTAG.20 JTAG.18 JTAG.16 JTAG.14 JTAG.12 JTAG.10 JTAG.8 JTAG.6 JTAG.4 31.11,82.55 26.99,82.55 v26.04,83.5 | U2.THERM 21.66,28.96 C16.1 | v24.13,70.17 25.08,69.22 v25.08,66.36 24.13,65.41 24.13,63.82 26.99,60.96 v28.26,60.96 | C38.2 v40.01,64.14 41.59,62.55 41.59,61.59 41.37,61.37 R28.1 | R28.1 C22.2 39.91,59.74 C13.2 | C13.2 37.37,57.2 R42.2 | C13.2 40.56,56.92 C42.2 | v42.86,60.64 41.91,60.64 R28.1 | C15.2 v14.29,19.37 12.38,19.37 v9.53,16.51 SV1.2 | v33.34,16.51 v28.89,16.51 | v14.92,27.3 11.43,27.3 SV1.2 | SV1.2 SV1.1 SV1.3 | SV1.8 SV1.7 SV1.9 | SV1.22 SV1.21
  Bottom 1.016: X1.3 67.84,7.8 X1.1 71.12,9.07 71.12,21.59 76.83,27.3 76.83,34.29 SV2.6 SV2.5
  other vias: 21.59,28.89 58.1,15.88 57.15,15.88 56.2,15.88 58.1,14.92 57.15,14.92 66.04,22.86 66.99,22.86 65.09,23.81 66.04,23.81 66.99,23.81 59.69,73.98 46.99,47.62 47.62,46.99 48.26,46.35 47.31,26.99 48.26,26.99 48.26,27.94 47.31,22.86 48.58,22.86 43.81,33.66 42.55,33.66 43.81,32.38 43.81,36.83 43.81,38.1 42.55,36.83 62.55,84.77 60.01,88.27 3.81,82.23 11.43,88.9 16.19,81.28 9.53,17.78 10.79,16.51 5.08,9.53 76.2,9.84 36.51,9.84 42.86,9.84
  pour Bottom (isolate 0.406): 0,91.44 0,0 81.28,0 81.28,91.44
  pour Top (isolate 0.406): 0,91.44 0,0 81.28,0 81.92,92.08
GND1  (via drill 0.4)
  Top 0.305: C14.- RJ1.SHIELD1 RJ1.SHIELD0 27.3,12.83 v27.3,17.14 RJ1.GND
LED1
  Top 0.305: U2.3 26.6,28.64 28.57,26.67 28.57,24.13 33.34,19.37 Q5.1
LED2
  Top 0.305: U2.2 26.15,28.14 27.62,26.67 R6.1 28.45,23.3 30.16,21.59 30.16,19.41 Q4.1
MDC
  Top 0.305: U2.13 18.75,30.14 18.41,30.48 18.41,33.34 22.54,37.47 JP2.5 22.54,38.42 23.81,39.69 R21.1
MDIO
  Top 0.305: U2.12 20.34,34.31 21.91,35.88 22.86,35.88 23.81,36.83 23.81,38.42 25.08,39.69 JP2.8 25.08,42.42 R22.1
  Bottom 0.305: R23.2 23.81,35.52 23.81,39.05 JP2.8
N$1
  Top 0.305: R32.2 LED1.A 48.48,10.57 STAT_LED1.A
N$2
  Top 0.305: R33.2 LED2.A 55.78,10.57 STAT_LED2.A
N$3
  Top 0.305: CN1.VBUS 38.41,10.17 37.15,11.43 R41.1
N$4
  Top 0.305: LED3.A 20.13,83.53 R30.2
N$5
  Bottom 0.305: 64.85,15.19 64.77,15.26 D1.A
  Bottom 1.016: X1.2 64.85,15.19
N$6
  Top 0.305: C3.1
  Top 0.813: C3.1 C2.1 54.23,20.57 C4.+ 58.09,22.15 U1.4 U1.2 | R18.1 C3.1
N$7
  Top 0.305: R7.1 72.17,25.72 3.3V_LED.A
N$8  (via drill 0.4)
  Top 0.305: R44.1 R43.2 55.56,74.11 v55.56,73.98
  Bottom 0.305: v55.56,73.98 50.48,68.9 50.48,59.69 51.44,58.74 51.44,15.88 52.07,15.24 52.07,5.14 S1.1
N$9
  Top 0.305: CN1.ID 40.8,10.01 41.91,11.11 R24.1
N$10
  Top 0.406: R1.1 71.98,14.8 VIN_LED.A
N$11
  Top 0.305: CN1.D+ 40.01,11.94 R3.1
N$12
  Top 0.305: U2.24 22.84,24.28 R5.1
N$13
  Bottom 0.305: RJ1.G+ 14.22,3.43 R10.1
N$14
  Bottom 0.305: RJ1.Y+ 27.69,3.43 R11.1
N$27
  Top 0.305: Q4.3 32.12,8.62 29.21,5.71 19.37,5.71 16.95,3.3 RJ1.G-
N$28
  Top 0.305: Q5.3 36.56,17.51 33.02,13.97 33.02,8.26 29.84,5.08 26.67,5.08 25.02,3.43 RJ1.Y-
N$29
  Top 0.305: CN1.D- 39.2,11.79 R2.1
N$35
  Top 0.305: STM32.73 51.11,58.1 55.32,58.1 C19.1
N$36
  Top 0.305: STM32.49 36.2,49.1 36.2,47.94 37.19,46.95 C20.1
N$45
  Top 0.305: R34.1 R35.2 C7.2 24.57,72.52 Q2.1
NINT
  Top 0.305: U2.14 18.3,29.64 17.78,30.16 17.78,33.66 21.27,37.15 21.27,38.42 22.54,39.69 JP2.6 22.54,42.42 R20.1
NRST
  Top 0.305: U2.15 17.85,29.14 17.14,29.84 17.14,33.97 20,36.83 JP2.3 20,38.42 21.27,39.69 21.27,41.27 20.64,41.91 R13.1
  Bottom 0.305: R9.2 20,35.05 JP2.3
OSC_IN
  Top 0.305: STM32.12 32.37,70.48 30.16,70.48 29.53,71.12 29.53,71.94 C8.2 | R35.1 C8.2 | C8.2 29.4,74.42 Q2.2
OSC_OUT
  Top 0.305: R34.2 27.94,70.17 27.94,69.85 32.3,69.85 STM32.13
PA0/ADC123_IN0
  Top 0.305: STM32.23 30.62,64.45 26.35,64.45 25.72,65.09 12.7,65.09 11.11,63.5 8.26,63.5 SV1.29
PA1
  Top 0.305: STM32.24 30.55,63.82 26.99,63.82 26.04,62.87 26.04,49.21 22.23,45.4 R20.2
PA2
  Top 0.305: STM32.25 30.48,63.18 28.89,63.18 27.3,61.59 27.3,47.31 25.4,45.4 R22.2
PA3/ADC123_IN3  (via drill 0.4)
  Top 0.305: STM32.26 30.52,59.69 30.16,59.69 v29.84,60.01
  Bottom 0.305: v29.84,60.01 15.88,60.01 13.65,62.23 SV1.28
PA4/ADC12_IN4  (via drill 0.4)
  Top 0.305: STM32.29 30.42,57.47 v29.84,57.47
  Bottom 0.305: v29.84,57.47 16.83,57.47 13.34,60.96 8.26,60.96 SV1.27
PA5/ADC12_IN5  (via drill 0.4)
  Top 0.305: STM32.30 30.18,56.52 v28.89,56.52
  Bottom 0.305: v28.89,56.52 16.19,56.52 13.02,59.69 SV1.26
PA6/ADC12_IN6  (via drill 0.4)
  Top 0.305: STM32.31 29.93,55.56 v29.53,55.56
  Bottom 0.305: v29.53,55.56 15.56,55.56 12.7,58.42 8.26,58.42 SV1.25
PA7
  Top 0.305: STM32.32 28.57,53.5 28.57,46.99 26.99,45.4 R12.2
PA8  (via drill 0.4)
  Top 0.305: STM32.67 53.86,51.12 57.15,51.12 58.42,52.39 61.91,52.39 v62.87,51.44
  Bottom 0.305: v62.87,51.44 64.14,50.16 64.14,46.67 68.9,41.91 SV2.11
PA13/TMS  (via drill 0.4)
  Top 0.305: 57.15,57.47 R37.1 57.25,57.37 57.47,57.15 | STM32.72 51.36,57.15 57.47,57.15 | 57.47,57.15 58.42,57.15 60.96,59.69 v60.96,61.59 | v62.87,69.53 66.99,73.66 66.99,81.28 64.77,83.5 57.47,83.5 56.52,82.55 v55.24,82.55
  Bottom 0.305: v60.96,61.59 60.96,67.63 v62.87,69.53 | v55.24,82.55 38.73,82.55 JTAG.7
PA14/TCK  (via drill 0.4)
  Top 0.305: STM32.76 51.62,63.82 55.24,63.82 v55.56,64.14 55.88,64.14 R51.2 | v61.91,70.48 66.36,74.93 66.36,80.96 64.45,82.87 58.1,82.87 v56.52,81.28
  Bottom 0.305: v55.56,64.14 v61.91,70.48 | JTAG.9 41.27,80.01 55.24,80.01 v56.52,81.28
PA15/TDI  (via drill 0.4)
  Top 0.305: STM32.77 51.55,64.45 53.98,64.45 v55.56,66.04 56.52,66.04 R48.1 | v60.96,71.44 65.72,76.2 65.72,80.64 64.14,82.23 59.69,82.23 v57.78,80.33
  Bottom 0.305: v55.56,66.04 v60.96,71.44 | JTAG.5 36.83,79.38 56.83,79.38 v57.78,80.33
PB0/ADC12_IN8  (via drill 0.4)
  Top 0.305: STM32.35 34.98,57.78 v36.2,57.78
  Bottom 0.305: v36.2,57.78 34.61,56.2 31.75,56.2 30.16,54.61 14.92,54.61 12.38,57.15 SV1.24
PB1/ADC12_IN9  (via drill 0.4)
  Top 0.305: STM32.36 33.15,55.24 v32.7,55.24
  Bottom 0.305: v32.7,55.24 31.75,55.24 30.48,53.98 13.97,53.98 12.06,55.88 8.26,55.88 SV1.23
PB3/TDO
  Top 0.305: JTAG.13 45.85,80.52 R36.1 46.8,78.42 57.78,78.42 60.96,81.6 63.82,81.6 65.09,80.33 65.09,76.83 60.64,72.39 51,72.39 STM32.89
PB4/TRST
  Top 0.305: JTAG.3 32.38,79.88 32.29,79.79 | 32.29,79.79 R49.1 | STM32.90 50.93,73.03 60.33,73.03 64.45,77.15 64.45,80.01 63.5,80.96 61.59,80.96 58.42,77.79 38.42,77.79 36.51,79.69 32.38,79.69 32.29,79.79
PB5  (via drill 0.4)
  Top 0.305: STM32.91 51.75,74.56 v51.75,74.61
  Bottom 0.305: SV1.38 33.02,74.93 33.66,74.3 42.23,74.3 44.13,72.39 49.53,72.39 v51.75,74.61
PB6  (via drill 0.4)
  Top 0.305: STM32.92 50.16,73.66 50.16,74.3 v50.48,74.61
  Bottom 0.305: v50.48,74.61 48.9,73.03 44.45,73.03 42.55,74.93 34.29,74.93 33.02,76.2 8.26,76.2 SV1.39
PB7  (via drill 0.4)
  Top 0.305: STM32.93 49.21,73.43 v49.21,74.61
  Bottom 0.305: v49.21,74.61 48.26,73.66 44.77,73.66 42.86,75.56 34.92,75.56 33.02,77.47 SV1.40
PB8/I2C1_SCL  (via drill 0.4)
  Top 0.305: STM32.95 47.62,73.26 47.62,75.25 48.58,76.2 60.01,76.2 v62.87,79.06
  Bottom 0.305: v62.87,79.06 68.26,79.06 71.12,76.2 73.34,76.2 SV2.40 74.61,79.88 R45.2
PB9/I2C1_SDA  (via drill 0.4)
  Top 0.305: STM32.96 46.99,73.33 46.99,75.56 48.26,76.83 59.05,76.83 v62.23,80.01
  Bottom 0.305: v62.23,80.01 69.53,80.01 SV2.39 R39.2
PB10  (via drill 0.4)
  Top 0.305: STM32.47 33.97,48.29 33.97,46.35 v33.34,45.72
  Bottom 0.305: v33.34,45.72 32.38,44.77 17.46,44.77 11.43,38.73 11.43,35.56 10.16,34.29 SV1.6
PB11
  Top 0.305: STM32.48 35.56,49.17 35.56,46.67 33.66,44.77 R16.2
PB12
  Top 0.305: STM32.51 43.5,50.16 43.5,48.9 41.91,47.31 39.69,45.09 38.73,45.09 38.42,45.4 35.88,45.4 35.24,44.77 R19.2
PB13
  Top 0.305: STM32.52 44.13,50.23 44.13,48.58 42.23,46.67 39.81,44.26 R17.2
PB14  (via drill 0.4)
  Top 0.305: STM32.53 44.77,50.31 44.77,48.26 41.59,45.09 v41.59,44.77
  Bottom 0.305: v41.59,44.77 40.96,44.13 18.1,44.13 12.38,38.42 12.38,34.61 10.79,33.02 8.26,33.02 SV1.5
PB15  (via drill 0.4)
  Top 0.305: STM32.54 45.4,50.38 45.4,47.94 43.18,45.72 v43.18,44.77
  Bottom 0.305: v43.18,44.77 41.91,43.5 18.73,43.5 13.34,38.1 13.34,33.97 11.11,31.75 SV1.4
PC0/ADC123_IN10
  Top 0.305: STM32.15 32.15,68.58 10.79,68.58 SV1.32
PC1  (via drill 0.4)
  Top 0.305: STM32.16 32.4,67.63 v31.75,67.63 | v27.3,62.87 26.67,62.23 26.67,48.26 23.81,45.4 R21.2
  Bottom 0.305: v27.3,62.87 31.75,67.31 v31.75,67.63
PC2/ADC123_IN12
  Top 0.305: STM32.17 32.64,66.67 30.48,66.67 29.21,67.94 12.7,67.94 10.79,66.04 8.26,66.04 SV1.31
PC3/ADC123_IN13
  Top 0.305: STM32.18 32.57,66.04 30.16,66.04 28.89,67.31 13.65,67.31 11.11,64.77 SV1.30
PC4
  Top 0.305: STM32.33 29.21,53.43 29.21,46.04 28.57,45.4 R15.2
PC5
  Top 0.305: STM32.34 29.84,53.36 29.84,44.58 R14.2
PC6  (via drill 0.4)
  Top 0.305: STM32.63 53.57,48.58 58.74,48.58 v59.37,49.21
  Bottom 0.305: v59.37,49.21 59.37,45.09 67.63,36.83 SV2.7
PC7  (via drill 0.4)
  Top 0.305: STM32.64 52.69,50.16 52.7,50.16 53.66,49.21 58.1,49.21 59.05,50.16 v60.01,50.16
  Bottom 0.305: v60.01,50.16 60.64,49.53 60.64,45.4 67.94,38.1 73.34,38.1 SV2.8
PC8  (via drill 0.4)
  Top 0.305: STM32.65 53.71,49.85 57.78,49.85 59.05,51.12 60.33,51.12 v61.59,49.85
  Bottom 0.305: v61.59,49.85 61.91,49.53 61.91,45.72 68.26,39.37 SV2.9
PC9  (via drill 0.4)
  Top 0.305: STM32.66 53.78,50.48 57.47,50.48 58.74,51.75 60.96,51.75 v61.59,51.12
  Bottom 0.305: v61.59,51.12 63.18,49.53 63.18,46.04 68.58,40.64 73.34,40.64 SV2.12
PC10  (via drill 0.4)
  Top 0.305: STM32.78 51.79,65.41 v53.66,65.41 | v65.09,67.63 69.53,72.07 69.53,86.04 BOOT/USART3.1
  Bottom 0.305: v53.66,65.41 60.64,72.39 61.28,72.39 63.82,69.85 63.82,68.9 v65.09,67.63
PC11  (via drill 0.4)
  Top 0.305: STM32.79 52.04,66.36 v52.7,66.36 | v64.77,69.22 67.94,72.39 BOOT/USART3.2
  Top 0.406: R52.2 67.94,85.92 BOOT/USART3.2
  Bottom 0.305: v52.7,66.36 53.66,66.36 60.33,73.03 61.59,73.03 64.77,69.85 v64.77,69.22
PC12  (via drill 0.4)
  Top 0.305: STM32.80 48.16,63.18 47.31,63.18 v45.09,65.41
  Bottom 0.305: v45.09,65.41 45.09,68.26 39.69,73.66 8.26,73.66 SV1.37
PC13/STAT_LED1  (via drill 0.4)
  Top 0.305: STM32.7 36.2,70.19 v36.2,70.48 | v48.9,17.46 48.26,16.83 R32.1
  Bottom 0.305: v36.2,70.48 36.83,71.12 40.32,71.12 43.5,67.94 43.5,64.77 50.16,58.1 50.16,18.73 v48.9,17.46
PC14/STAT_LED2  (via drill 0.4)
  Top 0.305: STM32.8 35.24,70.44 v35.24,71.12 | v50.16,14.92 50.99,14.1 R33.1
  Bottom 0.305: v35.24,71.12 35.88,71.75 40.64,71.75 44.13,68.26 44.13,65.09 50.8,58.42 50.8,15.56 v50.16,14.92
PC15/STAT_LED3
  Top 0.305: STM32.9 33.97,71 33.97,72.07 34.61,72.71 34.61,76.83 33.66,77.79 21.59,77.79 18.73,80.64 18.73,81.15 R30.1
PD0
  Top 0.305: STM32.81 51.58,67.31 56.83,67.31 66.99,57.15 SV2.23
PD1
  Top 0.305: STM32.82 51.51,67.94 57.15,67.94 66.67,58.42 73.34,58.42 SV2.24
PD2
  Top 0.305: STM32.83 51.43,68.58 57.47,68.58 66.36,59.69 SV2.25
PD3
  Top 0.305: STM32.84 51.36,69.22 57.78,69.22 66.04,60.96 73.34,60.96 SV2.26
PD4
  Top 0.305: STM32.85 51.29,69.85 58.1,69.85 65.72,62.23 SV2.27
PD5
  Top 0.305: STM32.86 51.22,70.48 58.42,70.48 65.41,63.5 73.34,63.5 SV2.28
PD6
  Top 0.305: STM32.87 51.15,71.12 58.74,71.12 65.09,64.77 SV2.29
PD7
  Top 0.305: STM32.88 51.07,71.75 59.05,71.75 64.77,66.04 73.34,66.04 SV2.30
PD8
  Top 0.305: STM32.55 52.99,43.5 63.5,43.5 66.99,46.99 SV2.15
PD9
  Top 0.305: STM32.56 53.06,44.13 63.18,44.13 67.31,48.26 73.34,48.26 SV2.16
PD10
  Top 0.305: STM32.57 53.13,44.77 62.87,44.77 67.63,49.53 SV2.17
PD11
  Top 0.305: STM32.58 53.21,45.4 62.55,45.4 67.94,50.8 73.34,50.8 SV2.18
PD12
  Top 0.305: STM32.59 53.28,46.04 62.23,46.04 68.26,52.07 SV2.19
PD13
  Top 0.305: STM32.60 53.35,46.67 61.91,46.67 68.58,53.34 73.34,53.34 SV2.20
PD14
  Top 0.305: STM32.61 53.42,47.31 61.59,47.31 68.9,54.61 SV2.21
PD15
  Top 0.305: STM32.62 53.5,47.94 61.28,47.94 69.22,55.88 73.34,55.88 SV2.22
PE0  (via drill 0.4)
  Top 0.305: STM32.97 45.4,72.45 v45.4,74.93
  Bottom 0.305: v45.4,74.93 46.04,75.56 60.01,75.56 66.99,68.58 73.34,68.58 SV2.34
PE1  (via drill 0.4)
  Top 0.305: STM32.98 44.45,72.2 v44.45,75.88
  Bottom 0.305: v44.45,75.88 44.77,76.2 60.33,76.2 66.67,69.85 SV2.33
PE2  (via drill 0.4)
  Top 0.305: v25.4,63.82 25.4,50.16 20.64,45.4 R13.2 | STM32.1 38.1,72.53 38.1,72.71 v38.73,72.71
  Bottom 0.305: v25.4,63.82 26.35,63.82 35.56,73.03 38.42,73.03 v38.73,72.71
PE3  (via drill 0.4)
  Top 0.305: STM32.2 37.15,72.78 37.15,75.25 v38.42,76.52
  Bottom 0.305: v38.42,76.52 38.73,76.83 60.64,76.83 66.36,71.12 73.34,71.12 SV2.36
PE4  (via drill 0.4)
  Top 0.305: STM32.3 36.51,72.7 36.51,76.2 v37.47,77.15
  Bottom 0.305: v37.47,77.15 37.78,77.47 60.96,77.47 66.04,72.39 SV2.35
PE5  (via drill 0.4)
  Top 0.305: STM32.4 35.88,72.63 35.88,77.15 v36.51,77.79
  Bottom 0.305: v36.51,77.79 36.83,78.11 61.28,78.11 65.72,73.66 73.34,73.66 SV2.38
PE6  (via drill 0.4)
  Top 0.305: STM32.5 35.24,72.56 35.24,78.42 v35.56,78.74
  Bottom 0.305: v35.56,78.74 61.59,78.74 65.41,74.93 SV2.37
PE7  (via drill 0.4)
  Top 0.305: STM32.38 32.66,53.34 v31.43,53.34
  Bottom 0.305: v31.43,53.34 14.61,53.34 10.79,49.53 SV1.18
PE8  (via drill 0.4)
  Top 0.305: STM32.39 32.41,52.39 v30.8,52.39
  Bottom 0.305: v30.8,52.39 14.92,52.39 10.79,48.26 8.26,48.26 SV1.17
PE9  (via drill 0.4)
  Top 0.305: STM32.40 32.17,51.44 v31.43,51.44
  Bottom 0.305: v31.43,51.44 15.24,51.44 10.79,46.99 SV1.16
PE10  (via drill 0.4)
  Top 0.305: STM32.41 31.92,50.48 v30.8,50.48
  Bottom 0.305: v30.8,50.48 15.56,50.48 10.79,45.72 8.26,45.72 SV1.15
PE11  (via drill 0.4)
  Top 0.305: STM32.42 31.68,49.53 v31.43,49.53
  Bottom 0.305: v31.43,49.53 15.88,49.53 10.79,44.45 SV1.14
PE12  (via drill 0.4)
  Top 0.305: STM32.43 31.43,48.58 v30.8,48.58
  Bottom 0.305: v30.8,48.58 16.19,48.58 10.79,43.18 8.26,43.18 SV1.13
PE13  (via drill 0.4)
  Top 0.305: STM32.44 31.82,48.26 v31.75,47.62
  Bottom 0.305: v31.75,47.62 16.51,47.62 10.79,41.91 SV1.12
PE14  (via drill 0.4)
  Top 0.305: STM32.45 32.7,48.44 32.7,47.31 32.07,46.67 v31.11,46.67
  Bottom 0.305: v31.11,46.67 16.83,46.67 10.79,40.64 8.26,40.64 SV1.11
PE15  (via drill 0.4)
  Top 0.305: STM32.46 33.34,48.36 33.34,46.99 v32.07,45.72
  Bottom 0.305: v32.07,45.72 17.14,45.72 10.79,39.37 SV1.10
RESET
  Top 0.305: STM32.14 32.22,69.22 23.5,69.22 13.34,79.38 12.06,79.38 10.99,80.45 C1.2 R31.2 9.34,83.53 RESET.1 11.27,86.04 45.09,86.04 46.35,85.09 46.35,82.55 JTAG.15
RX_N
  Top 0.305: U2.22 21.84,20.06 22.86,19.04 RJ1.RD-
  Bottom 0.305: RJ1.RD- R27.2
RX_P
  Top 0.305: U2.23 22.34,20.21 24.13,18.42 24.13,16.51 23.5,15.88 20.32,15.88 RJ1.RD+
  Bottom 0.305: RJ1.RD+ 20.64,13.02 R26.2
RXD0
  Top 0.305: U2.8 22.34,32.5 23.18,33.34 25.72,33.34 27.62,35.24 JP2.9 27.62,38.42 28.89,39.69 28.89,42.42 R15.1
RXD1
  Top 0.305: U2.7 22.84,32.05 23.5,32.7 26.04,32.7 28.89,35.56 28.89,38.42 30.16,39.69 JP2.12 R14.1
RXER
  Top 0.305: U2.10 21.34,33.41 22.54,34.61 24.45,34.61 26.35,36.51 26.35,38.42 27.62,39.69 JP2.10
TX_N
  Top 0.305: U2.20 20.84,20.53 17.78,17.47 RJ1.TD-
  Bottom 0.305: RJ1.TD- 17.78,13.97 19.05,12.7 R25.2
TX_P
  Top 0.305: U2.21 21.34,20.38 19.05,18.09 19.05,16.51 18.41,15.88 17.78,15.88 RJ1.TD+
  Bottom 0.305: RJ1.TD+ 16.51,13.14 R8.2
TXD0  (via drill 0.4)
  Top 0.305: U2.17 16.94,28.14 15.88,29.21 15.88,34.61 17.46,36.2 JP2.1 | v36.2,41.27 35.24,42.23 R19.1
  Bottom 0.305: JP2.1 18.73,39.05 18.73,41.27 19.68,42.23 35.24,42.23 v36.2,41.27
TXD1  (via drill 0.4)
  Top 0.305: U2.18 16.49,27.64 15.24,28.89 15.24,38.1 JP2.2 | v37.78,41.27 36.83,42.23 R17.1
  Bottom 0.305: JP2.2 17.46,40.96 19.37,42.86 36.2,42.86 v37.78,41.27
TXEN  (via drill 0.4)
  Top 0.305: U2.16 17.39,28.64 16.51,29.53 16.51,34.29 18.73,36.51 18.73,39.05 JP2.4 | v34.61,41.27 33.66,42.23 R16.1
  Bottom 0.305: JP2.4 20,40.96 20.64,41.59 34.29,41.59 v34.61,41.27
USB_DET  (via drill 0.4)
  Top 0.305: STM32.68 52.66,53.02 53.34,53.02 v53.98,52.39 | R41.2 37.15,14.61 39.05,16.51 39.05,25.08 53.98,40.01 v53.98,40.32
  Bottom 0.305: v53.98,40.32 v53.98,52.39
USB_ID  (via drill 0.4)
  Top 0.305: STM32.69 52.73,53.66 v57.78,53.66 | R24.2 41.91,15.24 40.96,16.19 40.96,22.54 57.78,39.37 v58.42,39.37
  Bottom 0.305: v58.42,39.37 58.42,53.66 v57.78,53.66
USB_N  (via drill 0.4)
  Top 0.305: STM32.70 52.08,55.02 53.02,55.02 v53.02,54.63 | R2.2 38.73,14.52 39.78,15.56 39.78,23.91 55.97,40.1 v55.59,40.26
  Bottom 0.305: v53.02,54.63 53.02,55.02 55.47,55.02 55.97,54.52 55.97,40.1 v55.59,40.26
USB_P  (via drill 0.4)
  Top 0.305: STM32.71 52.33,55.47 53.02,55.47 v53.02,55.85 | R3.2 40.32,15.47 40.23,15.56 40.23,23.72 56.43,39.91 v56.78,39.77
  Bottom 0.305: v53.02,55.85 53.02,55.47 55.66,55.47 56.43,54.7 56.43,39.91 v56.78,39.77
VBAT  (via drill 0.4)
  Top 0.305: STM32.6 38.52,68.58 v39.69,68.58
  Bottom 0.305: v39.69,68.58 40.13,68.58 R38.2
VDDA  (via drill 0.4)
  Top 0.305: STM32.22 33.02,62.76 v33.02,61.59
  Bottom 0.305: v33.02,61.59 L3.2 34.54,61.37 R29.1 37.26,60.09 C13.1 38.47,61.18 C22.1
VDDA_PHY  (via drill 0.4)
  Top 0.305: U2.19 20.34,25.4 | 20.34,25.4 20.34,24.45 | 20.34,24.45 20.34,22.74 L1.1 | 20.34,24.45 20.18,24.29 C25.1 16.68,24.29 C26.1 | U2.1 25.06,27.64 26.04,26.67 v26.04,25.08 26.04,23.62 C29.1 | v19.37,25.4 20.34,25.4
  Top 0.406: L1.1 19.05,21.45 19.05,20.32 14.61,15.88 14.61,13.65 16.19,12.06 20.64,12.06 21.59,13.02 RJ1.P5
  Bottom 0.305: v26.04,25.08 21.56,25.08 | 21.56,25.08 C27.1 | 21.56,25.08 19.68,25.08 v19.37,25.4 | 21.59,10.67 R26.1 R25.1 R8.1 | 21.59,10.67 R27.1 | 21.59,10.67 RJ1.P5 20.32,15.88 RJ1.P4 20.32,18.16 C15.1
VDDCR
  Top 0.305: U2.6 24.77,30.14 | 24.77,30.14 27.85,30.14 C21.1 | C17.1 24.86,30.23 24.77,30.14
VIN
  Top 0.813: R40.1 77.47,16.51 79.69,18.73 79.69,26.04 76.52,29.21 SV2.2 SV2.1
  Bottom 0.305: D1.C 65.09,18.67 65.09,18.73
  Bottom 0.813: JP1.3 72.07,27.94 SV2.1
  Bottom 1.016: SV2.2 SV2.1 72.07,25.72 65.09,18.73
VREF+  (via drill 0.4)
  Top 0.305: STM32.21 33.94,62.55 v34.29,62.23
  Bottom 0.305: v34.29,62.23 35.56,62.23 36.2,62.87 36.51,62.87 36.93,62.45 R29.2 37.88,63.28 C28.1
VREF-  (via drill 0.4)
  Top 0.305: STM32.20 34.01,63.18 v35.24,63.18
  Bottom 0.305: v35.24,63.18 36.42,64.36 C28.2 37.66,64.77 38.1,64.77 40.1,62.77 R28.2
XTAL1
  Top 0.305: Q3.2 31.86,30.81 C12.2 R4.2 30.19,29.64 U2.5
XTAL2
  Top 0.305: Q3.1 31.86,26.51 C11.2 R4.1 30.37,27.94 29.84,27.94 28.64,29.14 U2.4

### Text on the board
tNames: PB6 | PB9 | PB7 | PB8 | PC12 | PE6 | PB5 | PE5 | +3.3V | PE4 | +3.3V | PE3 | GND | PE1 | GND | PE0 | PC2 | GND | PC0 | GND | PA0 | PD6 | PC3 | PD7 | PA4 | PD4 | PA3 | PD5 | PA6 | PD2 | PA5 | PD3 | PB1 | PD0 | PB0 | PD1 | GND | PD14 | GND | PD15 | +3.3V | PD12 | +3.3V | PD13 | PE8 | PD10 | PE7 | PD11 | PE10 | PD8 | PE9 | PD9 | PE12 | GND | PE11 | GND | PE14 | PA8 | PE13 | PC9 | GND | PC8 | PE15 | PC7 | GND | PC6 | GND | GND | PB14 | GND | PB10 | GND | GND | +3.3V | PB15 | +3.3V | GND | GND | 3.3V | VIN | VIN | GND | VIN
bNames: RX | TX | 3.3V | Gnd | USART3 | PB7 | I2C1 | PB8 | PB6 | PB9 | RX | SCL | TX | PB5 | SDA | PE5 | PC12 | USART1 | PE6 | +3.3V | PE3 | +3.3V | PE4 | GND | PE0 | GND | PE1 | PC0 | GND | PC2 | GND | ANALOG | PC3 | PD7 | PA0 | PD6 | PA3 | PD5 | PA4 | PD4 | PA5 | PD3 | PA6 | PD2 | PB0 | PD1 | PB1 | PD0 | GND | PD15 | GND | PD14 | +3.3V | PD13 | +3.3V | PD12 | PE7 | PD11 | PE8 | PD10 | PE9 | PD9 | PE10 | PD8 | PE11 | GND | PE12 | I2C3 | GND | PE13 | PC9 | PA8 | SCL | PE14 | SDA | PE15 | GND | GND | USART6 | PC8 | PC7 | GND | PC6 | RX | GND | TX | PB10 | GND | PB14 | GND | PB15 | +3.3V | GND | +3.3V | GND | GND | 3.3V | VIN | VIN | GND | VIN

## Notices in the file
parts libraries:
microbuilder: This work is placed in the public domain, and may be freely used for commercial and non-commercial work with the following conditions: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
